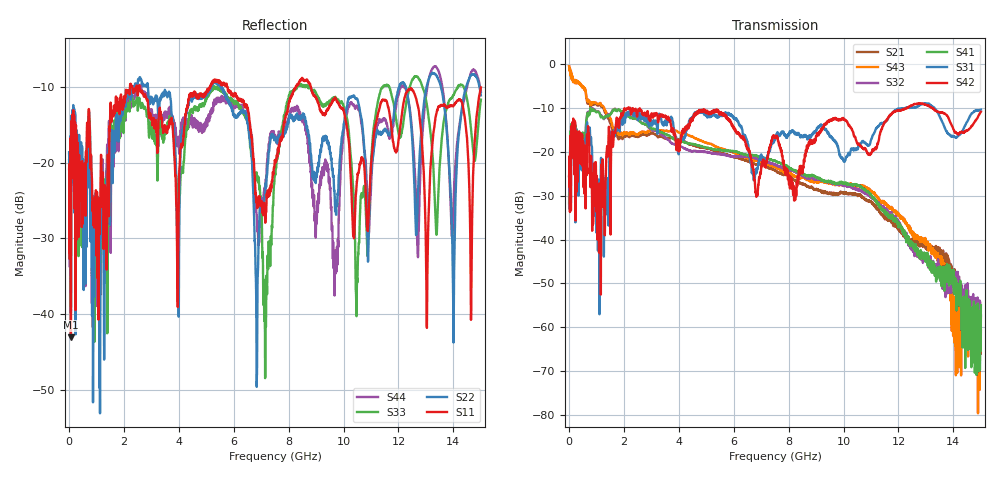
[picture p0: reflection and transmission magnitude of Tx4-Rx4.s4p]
! FILE: N:\QM 2007\Prüfprotokolle\Highspeed\Konfektionierte Ltg\L45593-D106\D30\8216\0002  kpl\IL  mit Chris Boards\Tx4-Rx4.s4p
# MHz S DB R 50.00
! FREQ  S11  S12  S13  S14
!  S21  S22  S23  S24
!  S31  S32  S33  S34
!  S41  S42  S43  S44
!  DB  ANG  DB  ANG  DB  ANG  DB  ANG
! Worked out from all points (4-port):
!   2999 points, 10 MHz to 15 GHz, reference 50 ohm
!   strongest paths, dB at 10 MHz, 3.755 GHz, 7.505 GHz, 11.26 GHz, 15 GHz:
!     S42: -25.5, -14.9, -16.9, -18.1, -10.9
!     S31: -25.7, -12.3, -17.3, -14.3, -10.4
!     S41: -31.8, -16.9, -22.0, -31.9, -54.9
!     S32: -30.2, -18.2, -23.0, -31.6, -57.4
!     S43: -0.5, -15.2, -23.4, -30.7, -60.6
!     S21: -0.6, -16.8, -24.2, -33.3, -57.2
!   lowest |S11| = -43.1 dB at 75 MHz (marker M1), VSWR 1.01, Z = 49.4 + j0.314 ohm
!   |S11| at or under -10 dB: 2.572 GHz to 5.145 GHz (2.573 GHz wide, 66.7 % of centre); 5.757 GHz to 8.265 GHz (2.508 GHz wide, 35.8 % of centre); 8.799 GHz to end of sweep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
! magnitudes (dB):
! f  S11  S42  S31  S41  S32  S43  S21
! 10 MHz  -20.9  -25.5  -25.7  -31.8  -30.2  -0.5  -0.6
! 75 MHz  -43.1  -33.4  -31.8  -19.4  -19.5  -1.7  -1.7
! 5.43 GHz  -9.4  -10.6  -11.8  -19.6  -20.5  -19.0  -20.1
! 6.835 GHz  -24.7  -30.1  -24.7  -20.9  -21.6  -22.0  -22.9
! 10.6 GHz  -20.2  -18.6  -18.3  -27.9  -28.7  -27.8  -30.0
! 13.99 GHz  -12.6  -14.8  -16.5  -46.9  -49.0  -53.2  -48.4
! 15 GHz  -10.1  -10.9  -10.4  -54.9  -57.4  -60.6  -57.2
